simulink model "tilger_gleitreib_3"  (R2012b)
settings: Solver=ode45  StartTime=0.0  StopTime=10.0  FixedStep=dt  MaxStep=dt  RelTol=1e-3
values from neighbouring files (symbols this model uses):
  ampl = 1    [diff_filter_1.m]    (also in foerd_gleit_1.m = 0.11; foerder_haft_gleit_1.m = 0.02; foerder_haft_gleit_2.m = 0.02; tilger_gleitreib3.m = 0.01)
  dt = 0.001    [coulomb_1.m]    (also in coulomb_10.m; coulomb_11.m; coulomb_2.m; coulomb_3.m)
  f = FG    (= 500)    [coulomb_5.m]    (also in dry_friction_1.m; feder_masse_1.m = logspace(e1,e2,5000); feder_masse_11.m = logspace(e1,e2,5000); feder_masse_12.m = logspace(e1,e2,5000))
  k = 10    [coulomb_10.m]    (also in coulomb_11.m; diff_filter_1.m = 250; diff_filter_2.m = 250; dry_friction_1.m = 2200)
  k1 = 5000    [feder_masse_1.m]    (also in feder_masse_11.m; feder_masse_13.m; feder_masse_14.m; tilger_gleitreib21.m)
  m = 400    [coulomb_1.m]    (also in coulomb_10.m = 10; coulomb_11.m = 10; coulomb_2.m; coulomb_3.m)
  m1 = 100    [feder_masse_1.m]    (also in feder_masse_11.m; feder_masse_13.m; feder_masse_14.m; position_reg_2.m = 1)
  rg = 20    [tilger_gleitreib1.m]    (also in tilger_gleitreib2.m = 100; tilger_gleitreib21.m = 0.5; tilger_gleitreib3.m = 8,      m1 = 0.1)
  x0 = [1;0]*1e-2    [rad_aufhaeng_1.m]    (also in slip_stick_3_1.m = 0.1; slip_stick_3_11.m = 0.1; suspension_1.m = [1 1 1 1]'; tilger_gleitreib1.m = 0.2)
libraries: simulink x2

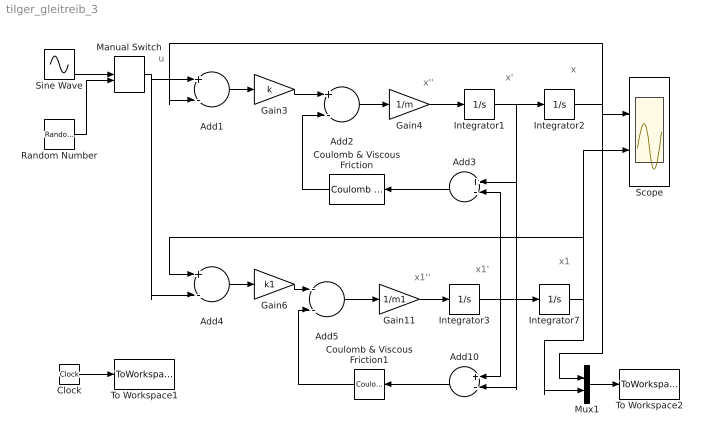
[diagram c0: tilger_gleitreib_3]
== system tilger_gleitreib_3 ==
  note: x1
  note: x1'
  note: x1''
  note: x''
  note: x'
  note: x
  note: u
  Add{1..4,10} (5 alike) : Sum  Inputs=+-
  Add5 : Sum  Inputs=--
  Clock : Clock
  Coulomb & Viscous Friction : simulink/Discontinuities/Coulomb & Viscous Friction  offset=[rg]  gain=0
  Coulomb & Viscous Friction1 : simulink/Discontinuities/Coulomb & Viscous Friction  offset=[rg]  gain=0
  Gain11 : Gain  Gain=1/m1
  Gain3 : Gain  Gain=k
  Gain4 : Gain  Gain=1/m
  Gain6 : Gain  Gain=k1
  Integrator1 : Integrator
  Integrator2 : Integrator  InitialCondition=x0
  Integrator3 : Integrator
  Integrator7 : Integrator
  Manual Switch : ManualSwitch
  Mux1 : Mux  Inputs=2
  Random Number : RandomNumber  Variance=0.01  SampleTime=dt
  Scope : Scope  NumInputPorts=2
  Sine Wave : Sin  Amplitude=ampl  Frequency=2*pi*f  SampleTime=0
  To Workspace1 : ToWorkspace  VariableName=t  SampleTime=-1
  To Workspace2 : ToWorkspace  VariableName=y  SampleTime=-1
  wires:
  Clock/1 -> To Workspace1/1
  Add1/1 -> Gain3/1
  Gain3/1 -> Add2/1
  Add2/1 -> Gain4/1
  Gain4/1 -> Integrator1/1
  Integrator1/1 -> Add10/2, Add3/1, Integrator2/1
  Integrator2/1 -> Scope/1, Mux1/1, Add1/2
  Add3/1 -> Coulomb & Viscous Friction/1
  Coulomb & Viscous Friction/1 -> Add2/2
  Add4/1 -> Gain6/1
  Gain6/1 -> Add5/1
  Add5/1 -> Gain11/1
  Gain11/1 -> Integrator3/1
  Integrator3/1 -> Add3/2, Add10/1, Integrator7/1
  Add10/1 -> Coulomb & Viscous Friction1/1
  Coulomb & Viscous Friction1/1 -> Add5/2
  Mux1/1 -> To Workspace2/1
  Integrator7/1 -> Mux1/2, Scope/2, Add4/1
  Manual Switch/1 -> Add4/2, Add1/1
  Sine Wave/1 -> Manual Switch/1
  Random Number/1 -> Manual Switch/2
